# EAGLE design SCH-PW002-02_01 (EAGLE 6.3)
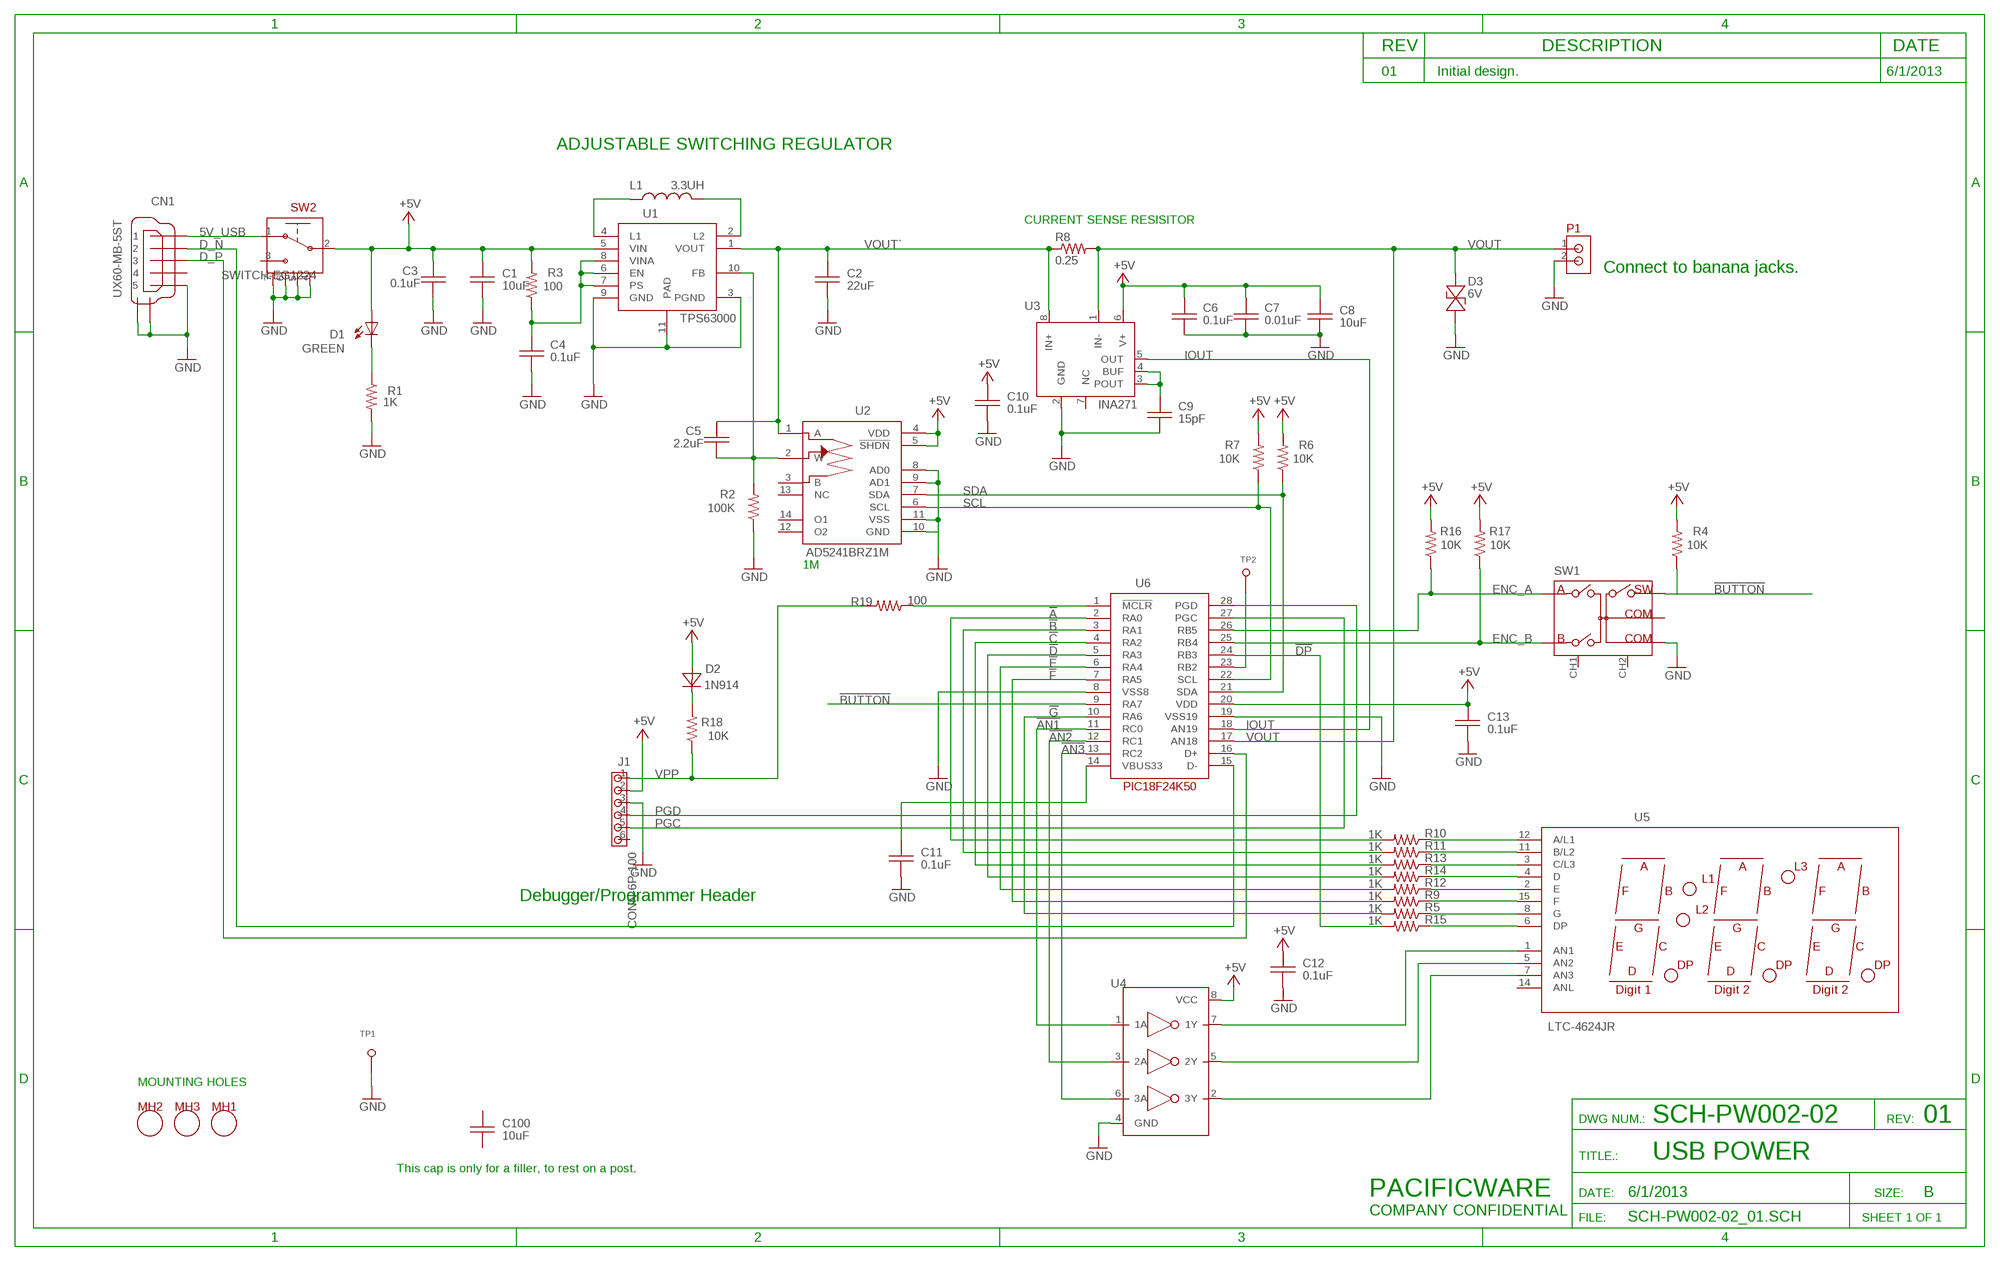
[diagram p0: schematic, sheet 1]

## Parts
C1  10uF  CAP-0805  [C0805]
C2  22uF  CAP-0805  [C0805]
C3  0.1uF  CAP0603  [C0603]
C4  0.1uF  CAP0603  [C0603]
C5  2.2uF  CAP0603  [C0603]
C6  0.1uF  CAP0603  [C0603]
C7  0.01uF  CAP0603  [C0603]
C8  10uF  CAP-0805  [C0805]
C9  15pF  CAP0603  [C0603]
C10  0.1uF  CAP0603  [C0603]
C11  0.1uF  CAP0603  [C0603]
C12  0.1uF  CAP0603  [C0603]
C13  0.1uF  CAP0603  [C0603]
C100  10uF  CAP-0805  [C0805]
CN1  UX60-MB-5ST  [UX60-MB-5ST]
D1  GREEN  LED-T1  [LED_T1]
D2  1N914  DIODE-SOD323  [SOD323F]
D3  6V  TVS  [C0603]
J1  CONN-6P-100  [CONN-6P-100]
L1  3.3UH  IND  [5045]
MH1  HOLE_MTG_125NP  [HOLE_125NP]
MH2  HOLE_MTG_125NP  [HOLE_125NP]
MH3  HOLE_MTG_125NP  [HOLE_125NP]
P1  CONN-2P-2.5MM  [CONN-2P-2_5MM]
R1  1K  RES0603  [R0603]
R2  100K  RES0603  [R0603]
R3  100  RES0603  [R0603]
R4  10K  RES0603  [R0603]
R5  1K  RES0603  [R0603]
R6  10K  RES0603  [R0603]
R7  10K  RES0603  [R0603]
R8  0.25  RES1206  [R1206]
R9  1K  RES0603  [R0603]
R10  1K  RES0603  [R0603]
R11  1K  RES0603  [R0603]
R12  1K  RES0603  [R0603]
R13  1K  RES0603  [R0603]
R14  1K  RES0603  [R0603]
R15  1K  RES0603  [R0603]
R16  10K  RES0603  [R0603]
R17  10K  RES0603  [R0603]
R18  10K  RES-0603  [R0603]
R19  100  RES0603  [R0603]
SW1  ENCODER_EVEJB  [ENCODER_EVJB]
SW2  SWITCH-EG1224  [SWITCH-EG1224]
TP1  TP_039  [HOLE_039_P]
TP2  TP_039  [HOLE_039_P]
U1  TPS63000  TPS6300X  [QFN10-5X2]
U2  AD5241BRZ1M  AD5241  [SOIC14]
U3  INA271  INA27X  [SOIC08]
U4  743G04  [SO8-MINI]
U5  LTC-4624JR  [LTC-4624JR]
U6  PIC18F24K50  [SSOP28]

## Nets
5V_USB [20mil]: CN1.1 SW2.1
!A: R10.2 U6.2(RA0)
!AN1: U4.1(1A) U6.11(RC0)
!AN2: U4.3(2A) U6.12(RC1)
!AN3: U4.6(3A) U6.13(RC2)
!B: R11.2 U6.3(RA1)
!BUTTON: R4.1 SW1.SW U6.9(RA7)
!C: R13.2 U6.4(RA2)
!D: R14.2 U6.5(RA3)
!DP: R15.2 U6.24(RB3)
!E: R12.2 U6.6(RA4)
!F: R9.2 U6.7(RA5)
!G: R5.2 U6.10(RA6)
+5V [20mil]: C1.1 C3.1 C6.1 C7.1 C8.1 C10.1 C12.1 C13.1 D1.1(A) D2.A J1.2 R3.2 R4.2 R6.2 R7.2 R16.2 R17.2 SW2.2 U1.5(VIN) U2.4(VDD) U2.5(!SHDN) U3.6(V+) U4.8(VCC) U6.20(VDD)
D_N: CN1.2 U6.15(D-)
D_P: CN1.3 U6.16(D+)
ENC_A: R16.1 SW1.A U6.26(RB5)
ENC_B: R17.1 SW1.B U6.25(RB4)
GND: C1.2 C2.2 C3.2 C4.2 C6.2 C7.2 C8.2 C9.2 C10.2 C11.2 C12.2 C13.2 CN1.5 CN1.6 CN1.7 D3.2 J1.3 P1.2 R1.2 R2.1 SW1.COM2 SW2.4 SW2.5 SW2.6 SW2.7 TP1.1 U1.3(PGND) U1.9(GND) U1.11(PAD) U2.8(AD0) U2.9(AD1) U2.10(GND) U2.11(VSS) U3.2(GND) U4.4(GND) U6.8(VSS8) U6.19(VSS19)
IOUT: U3.5(OUT) U6.18(AN19)
N$2: L1.2 U1.2(L2)
N$3: L1.1 U1.4(L1)
N$4: D2.K(C) R18.2
N$5: R10.1 U5.12(A/L1)
N$6: R11.1 U5.11(B/L2)
N$7: R13.1 U5.3(C/L3)
N$8: R14.1 U5.4(D)
N$9: R12.1 U5.2(E)
N$10: R9.1 U5.15(F)
N$11: R5.1 U5.8(G)
N$12: R15.1 U5.6(DP)
N$13: C5.2 R2.2 U1.10(FB) U2.2(W)
N$14: TP2.1 U6.23(RB2)
N$15: R19.1 U6.1(!MCLR)
N$16: C9.1 U3.3(POUT) U3.4(BUF)
N$17: C11.1 U6.14(VBUS33)
N$22: C4.1 R3.1 U1.6(EN) U1.7(PS) U1.8(VINA)
N$23: D1.2(C) R1.1
N$29: U4.7(1Y) U5.1(AN1)
N$30: U4.5(2Y) U5.5(AN2)
N$31: U4.2(3Y) U5.7(AN3)
PGC: J1.5 U6.27(PGC)
PGD: J1.4 U6.28(PGD)
SCL: R7.1 U2.6(SCL) U6.22(SCL)
SDA: R6.1 U2.7(SDA) U6.21(SDA)
VOUT [20mil]: D3.1 P1.1 R8.2 U3.1(IN-) U6.17(AN18)
VOUT` [20mil]: C2.1 C5.1 R8.1 U1.1(VOUT) U2.1(A) U3.8(IN+)
VPP: J1.1 R18.1 R19.2
Unconnected: C100.1 C100.2 CN1.4 J1.6 SW1.CH1 SW1.CH2 SW1.COM1 SW2.3 U2.3(B) U2.12(O2) U2.13(NC) U2.14(O1) U3.7(NC) U5.14(ANL)

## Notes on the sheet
- REV | DESCRIPTION | DATE
- 01 | Initial design. | 6/1/2013
- ADJUSTABLE SWITCHING REGULATOR
- CURRENT SENSE RESISITOR
- Connect to banana jacks.
- 1M
- Debugger/Programmer Header
- MOUNTING HOLES
- DWG NUM.: | SCH-PW002-02 | REV: | 01
- TITLE.: | USB POWER
- This cap is only for a filler, to rest on a post.
- PACIFICWARE | DATE: | 6/1/2013 | SIZE: | B
- COMPANY CONFIDENTIAL
- FILE: | SCH-PW002-02_01.SCH | SHEET 1 OF 1

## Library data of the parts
C1 C2 C8 C100 = Pacificware:CAP-0805
C3-C7 C9-C13 = Pacificware:CAP
CN1 = Pacificware:UX60-MB-5ST
D1 = Pacificware:LED-T1
D2 = Pacificware:DIODE-SOD323
D3 = Pacificware:TVS
J1 = Pacificware:CONN-6P-100
L1 = Pacificware:IND
MH1-MH3 = Pacificware:HOLE_MTG_125NP
P1 = Pacificware:CONN-2P-2.5MM
R1-R17 R19 = Pacificware:RES
R18 = Pacificware:RES-0603
SW1 = Pacificware:ENCODER_EVEJB
SW2 = Pacificware:SWITCH-EG1224
TP1 TP2 = Pacificware:TP_039
U1 = Pacificware:TPS6300X
U2 = Pacificware:AD5241
U3 = Pacificware:INA27X
U4 = Pacificware:743G04
U5 = Pacificware:LTC-4624JR
U6 = Pacificware:PIC18F24K50

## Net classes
1 20mil: width 0.508 mm

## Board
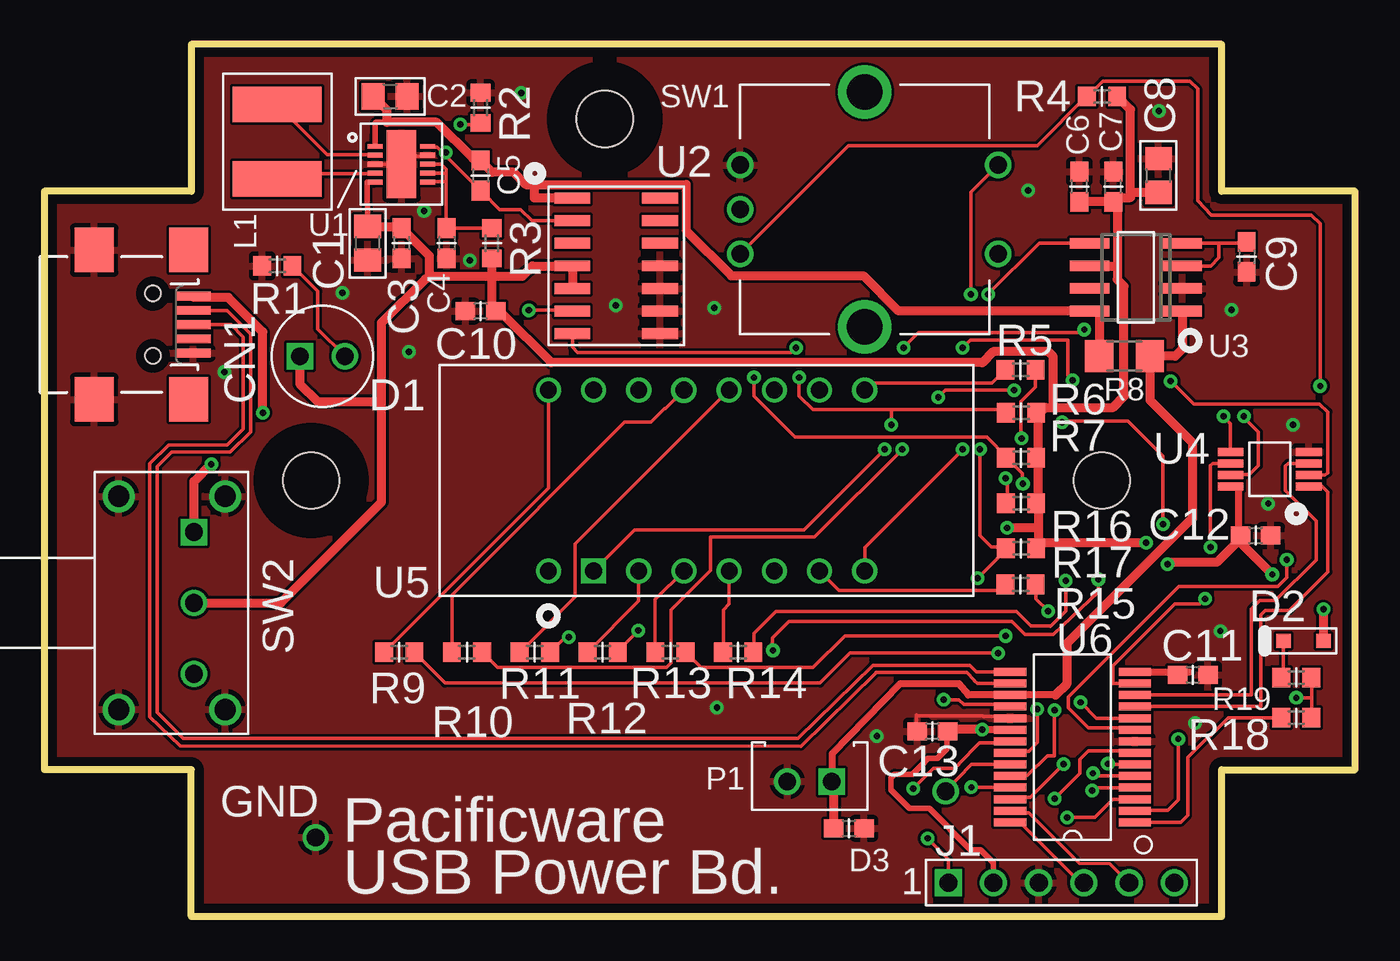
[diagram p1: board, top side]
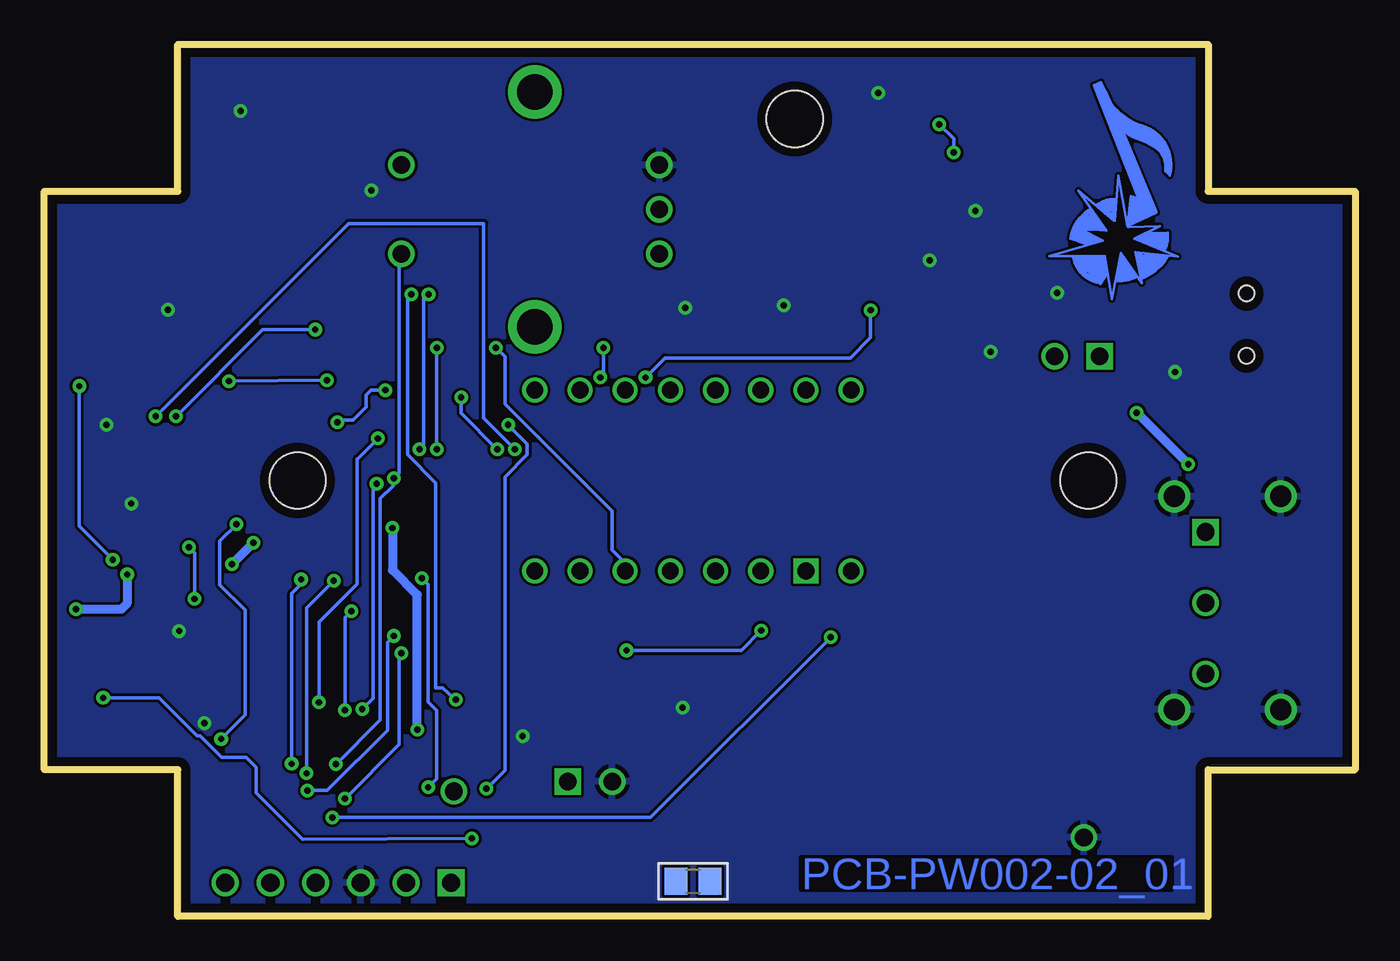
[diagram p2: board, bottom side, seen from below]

Size 73.66 x 49.02 mm. Coordinates in mm from the lower left corner, seen from the top.
Outline: 8.26,0 66.17,0 66.17,8.26 73.66,8.26 73.66,40.77 66.17,40.77 66.17,49.02 8.26,49.02 8.26,40.77 0,40.77 0,8.26 8.26,8.26 8.26,0
Copper layers (1*16): Top 0.0178mm / dielectric 59mil / Bottom 0.0178mm
Design rules "SSC-EAGLE-2Lyr_v1.0.0.3": minimum track width 6mil, minimum drill 14mil, track to track 6mil, track to pad 6mil, pad to pad 6mil, via to via 6mil, smd to smd 6mil, copper to edge 20mil, drill to drill 16mil, minimum pad ring 8mil, minimum via ring 8mil, stop-mask expansion 3mil, vias tented up to drill 0mil, thermal gap 10mil

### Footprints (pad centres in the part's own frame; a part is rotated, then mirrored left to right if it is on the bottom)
C0805 = smd 1.3 x 1.5: 1 -0.95,0; 2 0.95,0
C0603 = smd 1.1 x 1: 1 -0.85,0; 2 0.85,0
UX60-MB-5ST = smd 2 x 0.5: 1 2.25,1.6; 2 2.25,0.8; 3 2.25,0; 4 2.25,-0.8; 5 2.25,-1.6 | smd 2.2 x 2.5: 6 -3.3,-4.2; 7 -3.3,4.2; 8 2,4.2; 9 2,-4.2 | hole 0.889: 0,1.753; 0,-1.753
LED_T1 = drill 0.991 square: 1 0,0 | drill 0.991: 2 2.54,0
SOD323F = smd 0.8 x 0.8: A 1.125,0; K -1.125,0
CONN-6P-100 = drill 1.016 square: 1 0,0 | drill 1.016: 2 2.54,0; 3 5.08,0; 4 7.62,0; 5 10.16,0; 6 12.7,0
5045 = smd 2 x 5: 1 -2.1,0; 2 2.1,0
HOLE_125NP = hole 3.175: 0,0
CONN-2P-2_5MM = drill 0.991 square: 1 -1.25,0 | drill 0.991: 2 1.25,0
R0603 = smd 1 x 1.1: 1 -0.85,0; 2 0.85,0
R1206 = smd 1.6 x 1.803: 1 -1.422,0; 2 1.422,0
ENCODER_EVJB = drill 1: A -2.5,-7.5; B 2.5,-7.5; COM1 0,7; COM2 2.5,7; SW -2.5,7 | drill 2: CH1 -6.6,0; CH2 6.6,0
SWITCH-EG1224 = drill 0.991 square: 1 -3.988,0 | drill 0.991: 2 0,0; 3 3.988,0 | drill 1.194: 4 -5.994,1.753; 5 5.994,1.753; 6 5.994,-4.242; 7 -5.994,-4.242
HOLE_039_P = drill 0.991: 1 0,0
QFN10-5X2 = smd 0.28 x 0.85: 1 -1,-1.475; 2 -0.5,-1.475; 3 0,-1.475; 4 0.5,-1.475; 5 1,-1.475; 6 1,1.475; 7 0.5,1.475; 8 0,1.475; 9 -0.5,1.475; 10 -1,1.475 | smd 3.8 x 1.65: 11 0,0
SOIC14 = smd 0.61 x 2.007: 1 0.635,1.346; 2 1.905,1.346; 3 3.175,1.346; 4 4.445,1.346; 5 5.715,1.346; 6 6.985,1.346; 7 8.255,1.346; 8 8.255,6.274; 9 6.985,6.274; 10 5.715,6.274; 11 4.445,6.274; 12 3.175,6.274; 13 1.905,6.274; 14 0.635,6.274
SOIC08 = smd 0.6 x 2.2: 1 -1.905,-2.6; 2 -0.635,-2.6; 3 0.635,-2.6; 4 1.905,-2.6; 5 1.905,2.6; 6 0.635,2.6; 7 -0.635,2.6; 8 -1.905,2.6
SO8-MINI = smd 0.45 x 1.45: 1 -0.975,-2.2; 2 -0.325,-2.2; 3 0.325,-2.2; 4 0.975,-2.2; 5 0.975,2.2; 6 0.325,2.2; 7 -0.325,2.2; 8 -0.975,2.2
LTC-4624JR = drill 0.94 square: 1 -6.35,0 | drill 0.94: 2 -3.81,0; 3 -1.27,0; 4 1.27,0; 5 3.81,0; 6 6.35,0; 7 8.89,0; 8 8.89,10.16; 11 1.27,10.16; 14 -6.35,10.16; 15 -8.89,10.16; P$1 -8.89,0; P$2 6.35,10.16; P$3 3.81,10.16; P$4 -3.81,10.16 | drill 0.955: 12 -1.27,10.16
SSOP28 = smd 0.45 x 1.82: 1 -4.225,-3.5; 2 -3.575,-3.5; 3 -2.925,-3.5; 4 -2.275,-3.5; 5 -1.625,-3.5; 6 -0.975,-3.5; 7 -0.325,-3.5; 8 0.325,-3.5; 9 0.975,-3.5; 10 1.625,-3.5; 11 2.275,-3.5; 12 2.925,-3.5; 13 3.575,-3.5; 14 4.225,-3.5; 15 4.225,3.5; 16 3.575,3.5; 17 2.925,3.5; 18 2.275,3.5; 19 1.625,3.5; 20 0.975,3.5; 21 0.325,3.5; 22 -0.325,3.5; 23 -0.975,3.5; 24 -1.625,3.5; 25 -2.275,3.5; 26 -2.925,3.5; 27 -3.575,3.5; 28 -4.225,3.5

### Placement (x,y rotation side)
C1  18.16,37.85 270 top
C2  19.43,46.1 0 top
C3  20.07,37.85 270 top
C4  22.61,37.85 270 top
C5  24.51,41.66 270 top
C6  58.17,41.02 90 top
C7  60.07,41.02 90 top
C8  62.61,41.66 90 top
C9  67.56,37.08 270 top
C10  24.51,34.04 180 top
C11  64.54,13.59 0 top
C12  68.07,21.41 0 top
C13  49.91,10.41 180 top
C100  37.21,1.98 0 bottom
CN1  6.1,33.27 0 top
D1  14.35,31.5 0 top
D2  70.76,15.49 0 top
D3  45.21,4.95 0 top
J1  50.8,1.91 0 top
L1  13.08,43.56 90 top
MH1  31.5,44.83 90 top
MH2  14.99,24.51 0 top
MH3  59.44,24.51 0 top
P1  43,7.59 180 top
R1  13.08,36.58 180 top
R2  24.51,45.47 270 top
R3  25.15,37.85 270 top
R4  59.44,46.1 0 top
R5  54.86,30.73 0 top
R6  54.89,28.32 0 top
R7  54.89,25.78 0 top
R8  60.71,31.5 0 top
R9  19.94,14.86 0 top
R10  23.75,14.86 0 top
R11  27.56,14.86 0 top
R12  31.37,14.86 0 top
R13  35.18,14.86 0 top
R14  38.99,14.86 0 top
R15  54.86,18.67 0 top
R16  54.89,23.24 0 top
R17  54.89,20.7 0 top
R18  70.36,13.44 180 top
R19  70.36,11.18 0 top
SW1  46.1,39.75 90 top
SW2  8.41,17.63 270 top
TP1  15.24,4.45 0 top
TP2  50.65,7.04 0 top
U1  20.07,42.29 270 top
U2  28.32,41.02 270 top
U3  61.34,35.94 90 top
U4  68.86,25.15 90 top
U5  37.21,19.43 0 top
U6  57.78,9.53 90 top
U$1  [NOTE-SM-BOTTOM]  13.21,38.61 0 top

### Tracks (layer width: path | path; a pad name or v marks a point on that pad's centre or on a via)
5V_USB  (via drill 0.36)
  Top 0.508: v12.27,28.32 12.27,32.87 10.34,34.8 8.41,34.8 8.36,34.85 CN1.1 | v9.37,25.43 8.41,24.46 SW2.1
  Bottom 0.508: v9.37,25.43 v12.27,28.32
!A  (via drill 0.36)
  Top 0.203: v48.21,26.26 43.28,21.34 37.44,21.34 37.44,19.46 35.2,17.22 35.2,14.25 34.95,13.99 25.48,13.99 24.61,14.86 R10.2 | v50.24,29.18 50.65,29.59 v54.51,29.59 | v57.2,27.79 57.28,27.86 60.88,27.86 62.87,25.88 v62.87,22.05 | U6.2 61.29,5.97 63.14,5.97 63.73,6.55 v63.73,9.98
  Bottom 0.203: v48.21,26.26 50.24,28.3 v50.24,29.18 | v57.2,27.79 57.2,27.91 56.31,27.91 55.58,28.65 55.58,29.31 55.3,29.59 v54.51,29.59 | v63.73,9.98 62.38,11.33 62.38,17.22 63.8,18.64 63.8,21.11 v62.87,22.05
!AN1
  Top 0.203: U6.11 68.38,11.81 68.38,16.97 68.61,17.2 69.95,17.2 72.14,19.38 72.14,23.85 71.82,24.17 U4.1
!AN2
  Top 0.203: 71.32,25.38 71.4,25.45 U4.3 69.9,25.48 69.75,25.32 69.75,23.95 71.48,22.23 71.48,20.04 69.19,17.75 68.3,17.75 67.84,17.3 67.84,12.47 61.29,12.47 U6.12
!AN3  (via drill 0.36)
  Top 0.203: 66.93,25.38 67,25.45 U4.6 65.65,25.47 65.53,25.35 v65.53,20.75 | v65.23,17.86 64.95,17.58 63.52,17.58 60.05,14.1 60.05,13.11 61.27,13.11 U6.13
  Bottom 0.203: v65.53,20.75 65.23,20.45 v65.23,17.86
!B  (via drill 0.36)
  Top 0.203: v29.46,15.7 29.26,15.7 28.42,14.86 R11.2 | U6.3 61.27,6.58 60.05,6.58 59.03,5.56 v57.48,5.56
  Bottom 0.203: v29.46,15.7 39.6,5.56 v57.48,5.56
!BUTTON  (via drill 0.36)
  Top 0.203: SW1.SW 39.12,37.26 45.19,43.33 55.8,43.33 58.57,46.1 R4.1 58.67,46.15 59.49,46.97 64.39,46.97 64.82,46.53 64.82,40.23 65.58,39.42 71.2,39.42 71.7,38.94 v71.7,29.82 | v69.83,20.07 69.83,19.05 69.32,18.54 63.75,18.54 57.56,12.34 57.56,11.73 58.67,10.62 61.16,10.62 61.27,10.52 U6.9
  Bottom 0.203: v69.83,20.07 71.7,21.95 v71.7,29.82
!C  (via drill 0.36)
  Top 0.203: v58.88,7.09 59.03,7.24 61.27,7.24 U6.4 | R13.2 36.04,14.86 36.91,13.99 43.2,13.99 44.98,15.77 v54.03,15.77
  Bottom 0.203: v58.88,7.09 57.76,7.09 54.38,10.46 54.38,15.42 v54.03,15.77
!D  (via drill 0.36)
  Top 0.203: v58.93,8.05 59.08,7.9 61.27,7.9 U6.5 | 39.85,14.86 R14.2 39.88,14.9 39.88,15.9 41.12,17.14 54.63,17.14 55.45,16.33 56.54,16.33 56.54,16.31 57.4,17.17 v57.4,18.87
  Bottom 0.203: v58.93,8.05 58.93,17.35 v57.4,18.87
!DP  (via drill 0.36)
  Top 0.203: v56.77,11.61 56.77,9.04 56.36,9.04 55.24,7.92 54.3,7.92 U6.24 | R15.2 55.73,18.67 55.73,17.86 v56.41,17.17
  Bottom 0.203: v56.77,11.61 56.77,16.82 v56.41,17.17
!E  (via drill 0.36)
  Top 0.203: v59.77,8.59 59.79,8.56 61.27,8.56 U6.6 | R12.2 32.23,14.86 32.23,14.94 v33.38,16.08 | v59.23,18.95 59.23,18.24 56.72,15.85 55.12,15.85 54.38,16.59 41.83,16.59 40.92,15.67 40.92,14.99 v40.95,14.96
  Bottom 0.203: v40.95,14.96 34.49,14.96 v33.38,16.08 | v59.77,8.59 59.77,18.16 59.23,18.69 v59.23,18.95
!F  (via drill 0.36)
  Top 0.203: U6.7 60.88,9.2 60.76,9.32 58.67,9.32 58.19,8.84 58.19,8.05 v56.77,6.63 | v53.59,14.81 45.26,14.81 43.59,13.13 22.52,13.13 R9.2
  Bottom 0.203: v56.77,6.63 53.72,9.68 53.72,14.68 v53.59,14.81
!G  (via drill 0.36)
  Top 0.203: v58.24,12.04 59.13,11.15 61.27,11.15 U6.10 | R5.2 55.7,29.77 54.89,28.96 54.89,26.9 v54.91,26.87
  Bottom 0.203: v58.24,12.04 58.22,12.06 58.22,16.56 56.08,18.69 56.08,25.73 56.06,25.73 v54.91,26.87
+5V  (via drill 0.36)
  Top 0.305: C1.1 18.14,41.29 U1.5 | 50.95,10.5 C13.1 50.72,10.38 50.72,9.42 50.19,8.89 49.66,8.89 49.48,8.71 49.48,8.69 48.79,8 47.78,8 47.57,7.8 47.57,7.11 48.62,6.07 49.73,6.07 52.05,3.76 52.6,3.76 53.34,3.02 J1.2 | 52.82,10.5 v52.7,10.52
  Top 0.381: 67.13,21.41 67.13,24.18 U4.8 | U6.20 52.82,10.5
  Top 0.508: U2.5 U2.4 27.43,36.58 26.85,35.99 25.2,35.99 25.15,35.94 | C1.1 18.16,38.79 19.99,38.79 C3.1 20.24,38.53 21.64,37.13 21.64,35.97 | 25.15,35.94 25.15,34.04 C10.1 25.7,33.93 28.5,31.14 52.7,31.14 53.31,31.75 56.41,31.75 56.69,31.47 56.69,28.63 | 25.15,35.94 25.15,35.97 | 25.15,35.97 R3.2 | 25.15,35.97 21.64,35.97 | 21.64,35.97 21.41,35.84 18.95,33.38 18.95,28.88 | C6.1 58.17,40.18 60.07,40.18 C7.1 | 61.04,40.72 61.04,40.41 60.2,40.41 C7.1 | 61.04,40.72 61.04,45.36 R4.2 | 61.04,40.72 C8.1 | 60.3,36.63 60.3,39.95 60.22,39.95 C7.1 | 60.3,36.63 60.3,35.81 60.68,35.43 60.68,29.23 60.07,28.63 56.69,28.63 | U3.6 60.25,36.58 60.3,36.63 | 50.88,10.41 C13.1 50.96,10.52 v52.7,10.52 | 55.85,21.84 55.85,23.24 R16.2 55.85,23.47 55.85,25.78 R7.2 55.85,26.01 55.85,28.32 R6.2 56.08,28.45 56.26,28.63 56.69,28.63 | 55.85,21.84 55.85,20.7 R17.2 56.08,21.01 v61.92,21.01 | v69.01,19.23 67.13,21.11 67.13,21.41 C12.1 66.93,20.95 65.89,19.91 63.22,19.91 v63.12,19.81 | 55.85,21.84 v54.1,21.84 | v71.88,17.27 D2.A | SW2.2 13.28,17.63 18.95,23.29 18.95,28.88 | D1.1 14.35,29.95 15.34,28.96 18.87,28.96 18.95,28.88
  Bottom 0.508: v69.01,19.23 69.01,17.6 69.34,17.27 v71.88,17.27 | v63.12,19.81 v61.92,21.01 | v54.1,21.84 54.1,19.48 52.7,18.09 v52.7,10.52 52.78,10.44
D_N
  Top 0.203: CN1.2 10.26,34.07 11.58,32.75 11.58,27.25 10.45,26.11 7.14,26.11 6.33,25.29 6.33,11.46 7.81,10.01 42.36,10.01 46.55,14.12 52,14.12 52.37,13.75 U6.15
D_P
  Top 0.203: CN1.3 10.48,33.27 11.18,32.58 11.18,27.41 10.28,26.52 6.98,26.52 5.92,25.46 5.92,11.22 7.64,9.6 42.53,9.58 46.73,13.7 46.74,13.72 51.83,13.72 52.27,13.28 52.27,13.26 52.43,13.1 U6.16
ENC_A  (via drill 0.36)
  Top 0.203: v54.03,24.64 54.13,24.64 54.13,23.24 R16.1 | v57.28,8.56 55.42,6.71 54.41,6.71 54.3,6.6 U6.26
  Bottom 0.203: SW1.A 53.62,37.24 53.62,36.63 53.72,36.52 53.72,24.94 v54.03,24.64 54.08,24.56 54.08,24.21 54.79,23.5 54.79,11.05 v57.28,8.56
ENC_B  (via drill 0.36)
  Top 0.203: v52.45,19.02 54.13,20.7 R17.1 54.08,20.78 53.21,20.78 52.58,21.41 v52.58,26.26 | v52.09,7.26 54.28,7.26 U6.25 | v52.07,34.98 52.07,40.72 SW1.B
  Bottom 0.203: v52.45,19.02 52.09,18.67 52.09,12.06 51.61,11.58 51.61,7.75 v52.09,7.26 | v52.07,34.98 52.35,34.7 52.35,26.49 v52.58,26.26
GND  (via drill 0.36)
  Top 0.203: U1.3 U1.11 20.14,42.34 20.55,42.75 | U1.9 21.54,42.77 21.51,42.75 20.6,42.75 20.07,43.28 | 48.97,10.42 C13.2 49.02,10.45 49.02,11.33 49.07,11.28 52.76,11.28 52.78,11.25 53.98,11.25 54.08,11.15 U6.19
  other vias: 10.11,30.61 16.74,35.05 20.47,31.75 37.64,34.21 32.11,34.37 55.3,40.82 62.64,45.29 66.73,34.11 70.18,27.64 66.09,16.05 64.67,10.87 23.9,36.88 68.78,23.22 21.34,39.67 37.8,11.73 46.79,10.13 26.8,46.3
  pour Bottom: -0.89,-0.89 67.06,-0.89 67.06,7.37 75.31,7.37 75.31,49.91 -0.89,49.91
  pour Top: -0.64,0 76.2,0 76.2,41.27 66.67,41.27 66.67,50.16 -0.64,49.53
IOUT  (via drill 0.36)
  Top 0.203: v53.03,34.98 55.91,37.85 U3.5 | U6.18 54.18,11.91 51.69,11.91 51.41,12.19 v50.55,12.19
  Bottom 0.203: v53.03,34.98 53.26,34.75 53.26,25.96 51.69,24.38 51.69,12.85 51.28,12.85 v50.55,12.19
N$2
  Top 0.203: U1.2 18.57,42.8 18.54,42.82 15.9,42.82 13.08,45.64 L1.2
N$3
  Top 0.203: U1.4 18.57,41.78 18.54,41.76 13.36,41.76 13.08,41.48 L1.1
N$4
  Top 0.203: D2.K 69.64,13.47 R18.2
N$5
  Top 0.203: U5.12 34.9,28.55 34.85,28.55 34.09,27.79 32.61,27.79 22.91,18.09 22.91,14.86 R10.1
N$6
  Top 0.203: R11.1 29.82,17.96 29.82,20.93 U5.11
N$7
  Top 0.203: 34.34,14.86 R13.1 34.33,17.82 U5.3
N$8
  Top 0.203: R14.1 38.15,14.86 38.15,17.25 38.48,17.58 U5.4
N$9
  Top 0.203: U5.2 33.4,17.73 R12.1
N$10
  Top 0.203: R9.1 28.32,24.08 U5.15
N$11
  Top 0.203: U5.8 46.51,30 53.26,30 R5.1
N$12
  Top 0.203: U5.6 44.65,18.34 53.67,18.34 R15.1
N$13  (via drill 0.36)
  Top 0.203: 22.47,42.86 C5.2 24.59,40.74 25.58,39.75 26.77,39.75 27.41,39.12 U2.2 | 22.47,42.86 22.07,43.26 21.59,43.26 21.57,43.28 U1.10 | v23.37,44.53 24.43,44.53 24.51,44.6 R2.2 | v22.55,42.95 22.47,42.86
  Bottom 0.203: v23.37,44.53 22.55,43.71 v22.55,42.95
N$14
  Top 0.203: U6.23 52.11,8.55 TP2.1
N$15
  Top 0.203: U6.1 63.88,5.31 64.26,5.69 64.26,8.94 65.48,10.16 65.53,10.16 66.55,11.18 R19.1
N$16
  Top 0.203: 66.09,37.85 U3.4 63.96,37.77 | 66.09,37.85 67.49,37.85 C9.1 | U3.3 65.56,36.58 66.02,37.03 66.02,37.77 66.09,37.85
N$17
  Top 0.203: U6.14 | 64.37,13.75 C11.1
  Top 0.381: U6.14 64.37,13.75
N$22
  Top 0.203: U1.6 22.53,41.3 22.58,41.35 | U1.7 22.58,41.78 | U1.8 22.3,42.29 22.58,42.01 22.58,41.78 | R3.1 C4.1 22.58,38.79 22.58,41.35 | 22.58,41.78 22.58,41.35
N$23
  Top 0.203: R1.1 13.95,36.58 15.37,35.15 15.37,33.02 D1.2
N$29  (via drill 0.36)
  Top 0.203: v47.22,26.26 42.7,21.74 33.17,21.74 U5.1 | v67.41,28.12 67.41,28.04 68.22,27.23 68.22,25.35 67.72,24.84 66.68,24.84 U4.7
  Bottom 0.203: v67.41,28.12 56.57,38.96 48.97,38.96 48.97,28.02 v47.22,26.26
N$30  (via drill 0.36)
  Top 0.203: v58.45,32.99 58.27,32.82 49.12,32.82 v48.28,31.98 | U4.5 66.66,27.73 v66.27,28.12
  Bottom 0.203: v66.27,28.12 61.39,32.99 v58.45,32.99 | v48.28,31.98 47.78,31.47 47.78,28.8 41.76,22.78 41.76,20.6 41.02,19.86 U5.5
N$31  (via drill 0.36)
  Top 0.203: v63.3,30.1 64.59,28.8 71.65,28.8 72.14,28.37 72.14,24.94 71.96,24.82 U4.2 | v51.61,31.98 52.05,32.41 57.53,32.41 57.53,30.4 v57.78,30.15 | v51.61,26.26 46.1,20.75 U5.7
  Bottom 0.203: v57.78,30.15 v63.3,30.1 | v51.61,26.26 v51.61,31.98
PGC
  Top 0.203: J1.5 59.89,2.97 58.17,3 55.32,5.84 54.41,5.84 54.3,5.94 U6.27
PGD
  Top 0.203: J1.4 58.22,1.91 54.82,5.3 U6.28 54.3,5.28
SCL  (via drill 0.36)
  Top 0.203: v39.88,30.3 39.88,29.26 42.19,26.95 52.96,26.95 54.13,25.78 R7.1 54.2,25.7 54.2,25.65 54.97,24.89 54.97,24.31 v54.99,24.33 | U6.22 54.38,9.3 55.32,9.3 55.8,9.78 v55.8,11.66 | U2.6 29.62,34.09 v27.23,34.09
  Bottom 0.203: v55.8,11.66 55.19,12.27 55.19,24.08 v54.99,24.33 | v39.88,30.3 38.79,31.39 28.37,31.39 27.23,32.54 v27.23,34.09
SDA  (via drill 0.36)
  Top 0.203: 47.6,28.5 43.18,28.5 42.42,29.26 v42.42,30.3 | 47.6,28.5 53.95,28.5 54.13,28.32 R6.1 | v42.24,31.98 41.96,31.7 29.97,31.7 29.67,32 U2.7 | 47.6,28.5 v47.6,27.64 | U6.21 54.28,9.84 54.2,9.75 52.55,9.75 51.38,8.59 51.38,8.56 51.16,8.33 49.96,8.33 v48.82,7.19
  Bottom 0.203: v42.42,30.3 42.24,30.48 v42.24,31.98 | v47.6,27.64 46.53,26.57 46.53,25.96 47.78,24.71 47.78,8.23 v48.82,7.19
VOUT
  Top 0.203: U6.17
  Top 0.381: 56.84,12.45 U6.17 51.92,12.45 51.41,13.08 48.08,13.08 44.27,9.14 44.27,7.62 P1.1
  Top 0.508: U3.1 63.94,31.89 63.55,31.5 R8.2 62.13,29.03 64.52,26.64 64.52,22.4 57.45,15.34 57.45,13.06 56.84,12.45 | D3.1 44.36,7.49 P1.1
VOUT`
  Top 0.305: U1.1 18.59,43.99 18.59,44.6 18.64,44.65 19.25,44.65
  Top 0.508: R8.1 59.28,34.04 U3.8 48.01,34.04 46.02,36.02 38.61,36.02 36.07,38.56 36.07,41.15 27.53,41.15 | R8.1 | C2.1 19.25,45.34 19.25,44.65 22.05,44.65 24.08,42.62 24.28,42.62 C5.1 24.51,42.49 25.17,41.83 26.36,41.83 27.05,41.15 27.53,41.15 | U2.1 27.53,40.39 27.53,41.15
VPP  (via drill 0.36)
  Top 0.203: R18.1 71.22,13.32 71.22,12.34 | 71.22,12.34 71.22,11.19 R19.2 | v70.36,12.29 71.17,12.29 71.22,12.34 | J1.1 50.8,3.23 v49.63,4.39
  Bottom 0.203: v70.36,12.29 67.21,12.29 65.08,10.16 64.92,10.16 63.7,8.94 62.33,8.94 61.77,8.38 61.77,6.96 59.16,4.34 v49.63,4.39

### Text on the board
Bottom: PCB-PW002-02_01
tPlace: GND | Pacificware | USB Power Bd.
Document: Radius 0.18 | Radius 0.08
